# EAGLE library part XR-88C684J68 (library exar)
QUAD UART
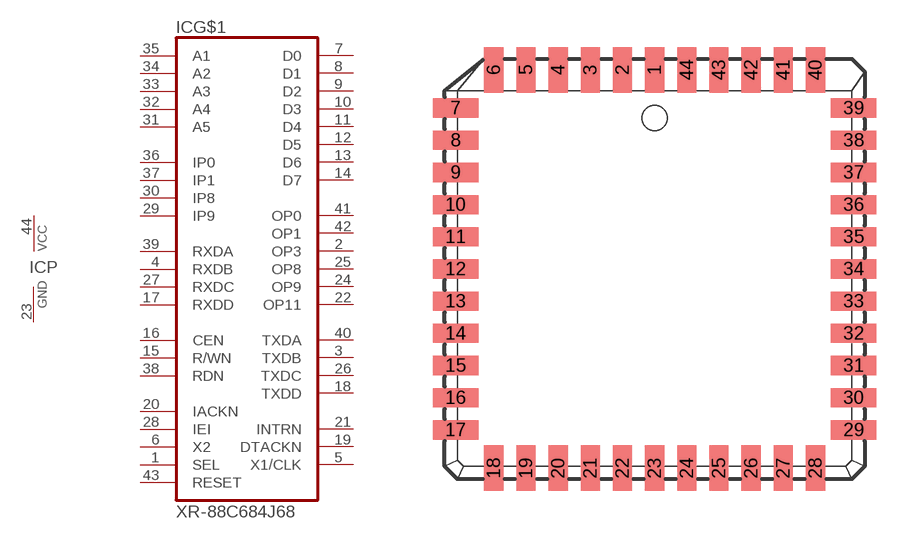
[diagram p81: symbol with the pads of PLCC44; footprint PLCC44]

Designator prefix IC; gates G$1=C684J68 P=PWRN

## XR-88C684J68 (OC_FARNELL: unknown; OC_NEWARK: unknown)  [PLCC44]
1  G$1:SEL  in
2  G$1:OP3  out
3  G$1:TXDB  out
4  G$1:RXDB  in
5  G$1:X1/CLK  out
6  G$1:X2  in
7  G$1:D0
8  G$1:D1
9  G$1:D2
10  G$1:D3
11  G$1:D4
12  G$1:D5
13  G$1:D6
14  G$1:D7
15  G$1:R/WN  in
16  G$1:CEN  in
17  G$1:RXDD  in
18  G$1:TXDD  out
19  G$1:DTACKN  out
20  G$1:IACKN  in
21  G$1:INTRN  out
22  G$1:OP11  out
23  P:GND  pwr
24  G$1:OP9  out
25  G$1:OP8  out
26  G$1:TXDC  out
27  G$1:RXDC  in
28  G$1:IEI  in
29  G$1:IP9  in
30  G$1:IP8  in
31  G$1:A5  in
32  G$1:A4  in
33  G$1:A3  in
34  G$1:A2  in
35  G$1:A1  in
36  G$1:IP0  in
37  G$1:IP1  in
38  G$1:RDN  in
39  G$1:RXDA  in
40  G$1:TXDA  out
41  G$1:OP0  out
42  G$1:OP1  out
43  G$1:RESET  in
44  P:VCC  pwr

## Footprint PLCC44 (pad centres in mm)
Plastic Leaded Chip Carrier
smd 0.76 x 1.8: 1 0,7.86; 2 -1.27,7.86; 3 -2.54,7.86; 4 -3.81,7.86; 5 -5.08,7.86; 6 -6.35,7.86; 18 -6.35,-7.86; 19 -5.08,-7.86; 20 -3.81,-7.86; 21 -2.54,-7.86; 22 -1.27,-7.86; 23 0,-7.86; 24 1.27,-7.86; 25 2.54,-7.86; 26 3.81,-7.86; 27 5.08,-7.86; 28 6.35,-7.86; 40 6.35,7.86; 41 5.08,7.86; 42 3.81,7.86; 43 2.54,7.86; 44 1.27,7.86
smd 1.8 x 0.76: 7 -7.86,6.35; 8 -7.86,5.08; 9 -7.86,3.81; 10 -7.86,2.54; 11 -7.86,1.27; 12 -7.86,0; 13 -7.86,-1.27; 14 -7.86,-2.54; 15 -7.86,-3.81; 16 -7.86,-5.08; 17 -7.86,-6.35; 29 7.86,-6.35; 30 7.86,-5.08; 31 7.86,-3.81; 32 7.86,-2.54; 33 7.86,-1.27; 34 7.86,0; 35 7.86,1.27; 36 7.86,2.54; 37 7.86,3.81; 38 7.86,5.08; 39 7.86,6.35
